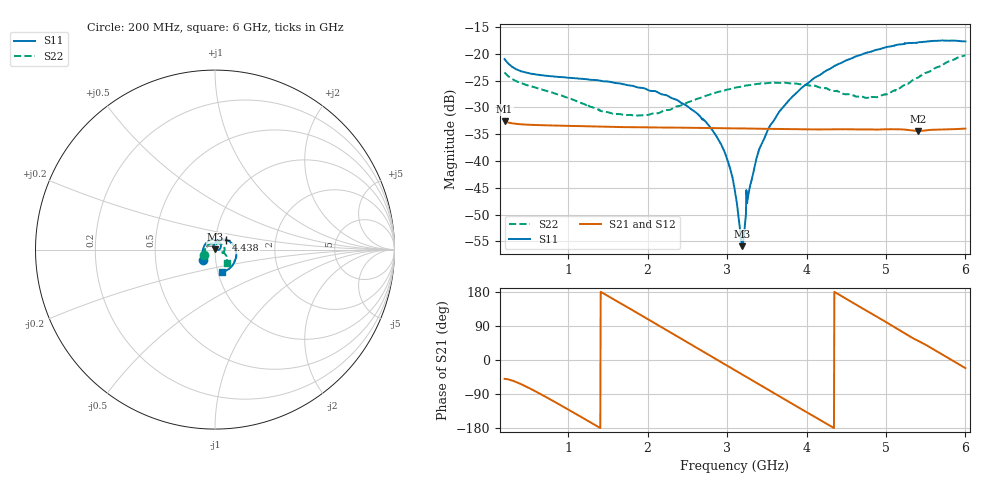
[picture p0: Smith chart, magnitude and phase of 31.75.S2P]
!Agilent Technologies,E5071C,MY46316741,A.11.02
!Date: Fri Apr 15 16:23:17 2022
!Data & Calibration Information:
!Freq	S11:SOLT2(ON)	S21:SOLT2(ON)	S12:SOLT2(ON)	S22:SOLT2(ON)
!PortZ  Port1:50+j0  Port2:50+j0
!Above PortZ is port z conversion or system Z0 setting when saving the data.
!When reading, reference impedance value at option line is always used.
# Hz S dB R 50
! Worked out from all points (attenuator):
!   1200 points, 200 MHz to 6 GHz, reference 50 ohm
!   highest |S21| = -32.59 dB at 200 MHz (marker M1); lowest = -34.4 dB at 5.405 GHz (marker M2)
!   lowest |S11| = -55.9 dB at 3.194 GHz (marker M3), VSWR 1.00, Z = 50.1 + j0.113 ohm
!   |S11| at or under -10 dB: start of sweep to end of sweep
!   |S22| runs from -31.5 to -20.3 dB; largest |S21 - S12| = 0.0001
!   S11 on the Smith chart (normalised r, x): 200 MHz: 0.87, -0.11; 4.438 GHz: 1.12, +0.12; 6 GHz: 1.05, -0.27
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2e8  -20.97 -137.9  -32.59 -49.6  -32.59 -49.6  -23.48 -151.7
4.757298e8  -23.54 177.2  -33.22 -70.6  -33.23 -70.6  -25.83 163.0
1.167473e9  -24.67 117.0  -33.50 -150.8  -33.51 -150.8  -29.19 106.3
1.578649e9  -25.41 86.5  -33.65 159.4  -33.65 159.5  -31.21 92.4
2.134946e9  -27.26 45.8  -33.76 91.6  -33.76 91.7  -31.07 82.8
2.497748e9  -29.75 17.6  -33.81 47.1  -33.81 47.2  -29.09 72.5
2.78799e9  -33.72 -3.4  -33.85 11.3  -33.85 11.4  -27.60 58.8
2.97181e9  -38.44 -14.3  -33.90 -11.3  -33.91 -11.2  -26.79 48.4
3.049208e9  -41.99 -16.8  -33.91 -20.8  -33.90 -20.7  -26.54 43.4
3.102419e9  -45.84 -11.3  -33.91 -27.3  -33.91 -27.2  -26.33 40.1
3.170142e9  -53.63 6.2  -33.92 -35.8  -33.93 -35.7  -26.16 35.7
3.194329e9  -55.91 45.0  -33.94 -38.7  -33.94 -38.6  -26.10 34.0
3.208841e9  -54.44 67.7  -33.93 -40.5  -33.94 -40.4  -26.04 33.0
3.271726e9  -46.04 115.9  -33.96 -48.2  -33.95 -48.2  -25.87 29.3
3.426522e9  -37.11 116.0  -33.99 -67.2  -33.99 -67.1  -25.50 19.0
3.673228e9  -30.51 99.1  -34.04 -97.5  -34.04 -97.4  -25.43 3.8
4.069892e9  -24.85 68.9  -34.11 -145.9  -34.12 -145.8  -25.96 -17.6
4.437531e9  -21.70 41.4  -34.08 169.0  -34.10 169.1  -27.31 -28.3
4.756797e9  -19.80 17.2  -34.13 129.9  -34.13 129.9  -28.24 -27.7
5.037364e9  -18.67 -3.4  -34.09 95.5  -34.09 95.6  -27.44 -22.3
5.405004e9  -17.87 -30.8  -34.41 50.5  -34.42 50.7  -24.43 -23.0
6e9  -17.68 -72.3  -33.96 -21.4  -33.97 -21.2  -20.27 -48.1
